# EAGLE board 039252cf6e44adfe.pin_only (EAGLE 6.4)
REV: A

Size 65 x 56.5 mm. Coordinates in mm from the lower left corner, seen from the top.
Outline: 0,36.45 3.68,36.45 arc-90 4.32,35.81 4.32,20.19 arc-90 3.68,19.56 0,19.56 0,19.68
Outline: 44.7,3.17 45.34,3.17 arc90 45.97,3.81 45.97,19.3 arc90 45.34,19.94 44.7,19.94 arc90 44.07,19.3 44.07,3.81 arc90 44.7,3.17
Copper layers (1*16): Top 0.035mm / dielectric 1.5mm / Bottom 0.035mm
Design rules "adafruit *": minimum track width 8mil, minimum drill 15.5mil, track to track 8mil, track to pad 8mil, pad to pad 8mil, via to via 8mil, smd to smd 8mil, copper to edge 10mil, drill to drill 8mil, minimum pad ring 10mil, minimum via ring 8mil, stop-mask expansion 2mil, vias tented up to drill 20mil, thermal gap 10mil
Milling: 2 lines

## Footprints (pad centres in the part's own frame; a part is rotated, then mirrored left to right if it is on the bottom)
1X25_ROUND_70MIL = drill 1 pad 1.676: 1 -30.48,0; 2 -27.94,0; 3 -25.4,0; 4 -22.86,0; 5 -20.32,0; 6 -17.78,0; 7 -15.24,0; 8 -12.7,0; 9 -10.16,0; 10 -7.62,0; 11 -5.08,0; 12 -2.54,0; 13 0,0; 14 2.54,0; 15 5.08,0; 16 7.62,0; 17 10.16,0; 18 12.7,0; 19 15.24,0; 20 17.78,0; 21 20.32,0; 22 22.86,0; 23 25.4,0; 24 27.94,0; 25 30.48,0
FIDUCIAL_1MM = smd 1 x 1: 1 0,0
0805-NO = smd 1.3 x 1.5: 1 -0.95,0; 2 0.95,0
PI_HAT_NOSLOTS = drill 0.9 pad 1.676: 1 8.37,51.23; 2 8.37,53.77; 3 10.91,51.23; 4 10.91,53.77; 5 13.45,51.23; 6 13.45,53.77; 7 15.99,51.23; 8 15.99,53.77; 9 18.53,51.23; 10 18.53,53.77; 11 21.07,51.23; 12 21.07,53.77; 13 23.61,51.23; 14 23.61,53.77; 15 26.15,51.23; 16 26.15,53.77; 17 28.69,51.23; 18 28.69,53.77; 19 31.23,51.23; 20 31.23,53.77; 21 33.77,51.23; 22 33.77,53.77; 23 36.31,51.23; 24 36.31,53.77; 25 38.85,51.23; 26 38.85,53.77; 27 41.39,51.23; 28 41.39,53.77; 29 43.93,51.23; 30 43.93,53.77; 31 46.47,51.23; 32 46.47,53.77; 33 49.01,51.23; 34 49.01,53.77; 35 51.55,51.23; 36 51.55,53.77; 37 54.09,51.23; 38 54.09,53.77; 39 56.63,51.23; 40 56.63,53.77 | hole 2.8: 3.5,3.5; 3.5,52.5; 61.5,52.5; 61.5,3.5
SOLDERJUMPER_CLOSEDWIRE = smd 1.168 x 1.6: 1 -0.762,0; 2 0.762,0 | smd 0.635 x 0.203: WIRE 0,0
SOIC8_150MIL = smd 0.6 x 2.2: 1 -1.905,-2.6; 2 -0.635,-2.6; 3 0.635,-2.6; 4 1.905,-2.6; 5 1.905,2.6; 6 0.635,2.6; 7 -0.635,2.6; 8 -1.905,2.6

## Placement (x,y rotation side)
CONN1  HEADER-1X25  [1X25_ROUND_70MIL]  32.77,47.24 0 top
FID2  FIDUCIAL""  [FIDUCIAL_1MM]  8.38,1.52 0 top
FID3  FIDUCIAL""  [FIDUCIAL_1MM]  58.42,49.53 0 top
R1  3.9K  [0805-NO]  54.48,1.27 180 top
R2  3.9K  [0805-NO]  56.01,5.33 90 top
R3  3.9K  [0805-NO]  50.67,1.27 0 top
RPI1  RASPBERRYPI_BPLUS_HATNOSLOTS  [PI_HAT_NOSLOTS]  0,0 0 top
SJ1  WP  [SOLDERJUMPER_CLOSEDWIRE]  47.12,1.27 0 top
U1  CAT24C32  [SOIC8_150MIL]  50.93,4.83 270 top
U$1  [ADAFRUIT_5MM]  0.51,7.24 0 top
U$2  [PIHATLOGO]  57.91,21.08 0 top
U$3  [PCBFEAT-REV-056]  2.54,16.26 0 top
U$5  [HAD_LOGO_200MIL]  6.1,20.19 0 top

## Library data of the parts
CONN1 R1-R3 RPI1 SJ1 U1 U$1-U$3 U$5 = microbuilder
FID2 FID3 = microbuilder; BOM: EXCLUDE

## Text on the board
tPlace: SDA | SCL | TXD | RXD | #4 | #17 | #18 | #27 | #22 | #23 | #24 | #25 | MOSI | MISO | CLK | CE0 | CE1 | #5 | #6 | #12 | #13 | #16 | #19 | #20 | #21 | +3V | GND | Hackaday Perma-Proto BLACK HAT! | +5V | GND | WP
tSilk: + | + | + | +

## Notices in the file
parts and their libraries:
microbuilder: This work is placed in the public domain, and may be freely used for commercial and non-commercial work with the following conditions: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
